| TEXAS INSTRUMENTS INCORPORATED
| Standard Linear and Logic Group
| IBIS Model of SN74ALVC16244A
| 16-BIT BUFFER/DRIVER WITH 3-STATE OUTPUTS
| This file contains package information for the following:
|  TSSOP 48-pin (DGG) package as [Component] ALVC16244A_DGG
|  SSOP 48-pin (DL) package as [Component] ALVC16244A_DL
|  jrBGA 48-pin (GQL) package as [Component] ALVC16244A_GQL
|  jrBGA 48-pin (GQL) package as [Component] ALVC16244A_ZQL
| This device can be powered at the following Vccs:
|  1.8 volt Vcc
|  2.5 volt Vcc
|  2.7 volt Vcc
|  3.3 volt Vcc
| This file provides unique models under the [Model Selector] for each Vcc.
| For operation at a specific Vcc, select the appropriate model after each
| [Model Selector] keyword.
[IBIS Ver]   3.2
[Comment char]  |_char
[File Name]   sn74alvc16244a.ibs
[File Rev]   1.1 | b_die
[Date]   June 26, 2007
[Source]   Data created from TI-SPICE simulations at TI-SLL.
[Notes]   The following is an IBIS list for the SN74ALVC16244A.
   Please contact sllibis@ti.com with questions and
   comments concerning SLL IBIS models.
   This IBIS model is created from a BA (back annotated netlist)
   - FILE REV HISTORY
   - 1.1 Release IBIS file on 05/28/07
[Disclaimer] Property of Texas Instruments Incorporated.  Unauthorized
   reproduction and/or distribution is strictly prohibited.
   This product is protected under copyright law.
   Created  2007, (C) Copyright  2007, Texas Instruments
   Incorporated, All Rights Reserved
   UNLESS THERE IS A SIGNED, WRITTEN AGREEMENT TO THE
   CONTRARY, TEXAS INSTRUMENTS (TI) IS PROVIDING THE IBIS
   MODELS  AND WITHOUT ANY WARRANTY, EXPRESSED OR
   IMPLIED.  TI assumes no liability for:
   1) the accuracy of the IBIS models provided to your
   company;
   2) the proper functioning of these IBIS Models in your
   design or for any resulting applications; or
   3) infringement of patents, copyrights or intellectual
   property rights resulting from your use of these IBIS
   models.
   TI provides IBIS Models as a service to our customers.
   You and your company shall not distribute, sell or give
   these models to anyone else without prior written
   permission from TI.
   TI reserves the right to make changes to our products or
   to discontinue any semiconductor product or service
   without notice, and advises our customers to obtain the
   latest version of relevant information to verify, before
   placing orders, that the information being relied on is
   current.
   Please be aware that your receipt and use of the IBIS
   information provided shall serve as acceptance of these
   terms and conditions.  If you do not accept these terms,
   you should return or destroy the IBIS models and any
   other accompanying information immediately.
| Component SN74ALVC16244A_DGG 48-PIN TSSOP
[Component]   SN74ALVC16244A_DGG
[Manufacturer]   Texas Instruments, Inc.
[Package]
|   typ   min   max
R_pkg   6.200e-02   5.000e-02   7.800e-02
L_pkg   3.527e-09   3.128e-09   4.255e-09
C_pkg   5.300e-13   4.170e-13   6.850e-13
[Pin]   signal_name   model_name   R_pin   L_pin   C_pin
1   N1OE   ALVC16244A_NOE   5.000e-02   4.250e-09   6.710e-13
2   1Y1   ALVC16244A_OUT   5.700e-02   3.956e-09   6.740e-13
3   1Y2   ALVC16244A_OUT   7.100e-02   3.922e-09   6.190e-13
4   GND   GND   7.800e-02   3.841e-09   6.180e-13
5   1Y3   ALVC16244A_OUT   5.600e-02   3.535e-09   5.550e-13
6   1Y4   ALVC16244A_OUT   5.800e-02   3.464e-09   5.030e-13
7   VCC   POWER   6.000e-02   3.362e-09   4.980e-13
8   2Y1   ALVC16244A_OUT   6.100e-02   3.293e-09   4.620e-13
9   2Y2   ALVC16244A_OUT   6.300e-02   3.240e-09   4.550e-13
10   GND   GND   6.300e-02   3.175e-09   4.420e-13
11   2Y3   ALVC16244A_OUT   6.400e-02   3.153e-09   4.290e-13
12   2Y4   ALVC16244A_OUT   6.500e-02   3.128e-09   4.180e-13
13   3Y1   ALVC16244A_OUT   6.500e-02   3.128e-09   4.180e-13
14   3Y2   ALVC16244A_OUT   6.400e-02   3.154e-09   4.290e-13
15   GND   GND   6.300e-02   3.174e-09   4.420e-13
16   3Y3   ALVC16244A_OUT   6.300e-02   3.241e-09   4.550e-13
17   3Y4   ALVC16244A_OUT   6.100e-02   3.293e-09   4.620e-13
18   VCC   POWER   6.000e-02   3.362e-09   4.970e-13
19   4Y1   ALVC16244A_OUT   5.800e-02   3.464e-09   5.030e-13
20   4Y2   ALVC16244A_OUT   5.600e-02   3.537e-09   5.600e-13
21   GND   GND   7.700e-02   3.839e-09   6.260e-13
22   4Y3   ALVC16244A_OUT   7.100e-02   3.917e-09   6.270e-13
23   4Y4   ALVC16244A_OUT   5.800e-02   3.955e-09   6.850e-13
24   N4OE   ALVC16244A_NOE   5.200e-02   4.255e-09   6.790e-13
25   N3OE   ALVC16244A_NOE   5.100e-02   4.254e-09   6.760e-13
26   4A4   ALVC16244A_IN   5.800e-02   3.957e-09   6.790e-13
27   4A3   ALVC16244A_IN   7.100e-02   3.920e-09   6.210e-13
28   GND   GND   7.800e-02   3.843e-09   6.220e-13
29   4A2   ALVC16244A_IN   5.600e-02   3.539e-09   5.600e-13
30   4A1   ALVC16244A_IN   5.800e-02   3.466e-09   5.030e-13
31   VCC   POWER   6.000e-02   3.363e-09   4.970e-13
32   3A4   ALVC16244A_IN   6.100e-02   3.294e-09   4.620e-13
33   3A3   ALVC16244A_IN   6.300e-02   3.241e-09   4.540e-13
34   GND   GND   6.300e-02   3.175e-09   4.410e-13
35   3A2   ALVC16244A_IN   6.400e-02   3.153e-09   4.290e-13
36   3A1   ALVC16244A_IN   6.500e-02   3.129e-09   4.170e-13
37   2A4   ALVC16244A_IN   6.500e-02   3.129e-09   4.170e-13
38   2A3   ALVC16244A_IN   6.400e-02   3.152e-09   4.290e-13
39   GND   GND   6.400e-02   3.176e-09   4.410e-13
40   2A2   ALVC16244A_IN   6.300e-02   3.241e-09   4.540e-13
41   2A1   ALVC16244A_IN   6.100e-02   3.293e-09   4.620e-13
42   VCC   POWER   6.000e-02   3.363e-09   4.970e-13
43   1A4   ALVC16244A_IN   5.800e-02   3.464e-09   5.030e-13
44   1A3   ALVC16244A_IN   5.600e-02   3.534e-09   5.610e-13
45   GND   GND   7.800e-02   3.841e-09   6.260e-13
46   1A2   ALVC16244A_IN   7.100e-02   3.920e-09   6.220e-13
47   1A1   ALVC16244A_IN   5.700e-02   3.955e-09   6.770e-13
48   N2OE   ALVC16244A_NOE   5.100e-02   4.252e-09   6.720e-13
| Component SN74ALVC16244A_DL 48-PIN SSOP
[Component]   SN74ALVC16244A_DL
[Manufacturer]   Texas Instruments, Inc.
[Package]
|   typ   min   max
R_pkg   4.800e-02   3.800e-02   5.300e-02
L_pkg   6.046e-09   5.084e-09   7.968e-09
C_pkg   8.130e-13   5.690e-13   1.157e-12
[Pin]   signal_name   model_name   R_pin   L_pin   C_pin
1   N1OE   ALVC16244A_NOE   4.600e-02   7.968e-09   1.017e-12
2   1Y1   ALVC16244A_OUT   4.400e-02   7.299e-09   1.157e-12
3   1Y2   ALVC16244A_OUT   4.300e-02   6.765e-09   1.058e-12
4   GND   GND   4.100e-02   6.269e-09   9.330e-13
5   1Y3   ALVC16244A_OUT   3.800e-02   5.856e-09   8.290e-13
6   1Y4   ALVC16244A_OUT   4.600e-02   5.802e-09   7.900e-13
7   VCC   POWER   5.000e-02   5.656e-09   7.380e-13
8   2Y1   ALVC16244A_OUT   5.300e-02   5.500e-09   6.430e-13
9   2Y2   ALVC16244A_OUT   5.200e-02   5.304e-09   6.060e-13
10   GND   GND   5.300e-02   5.189e-09   5.830e-13
11   2Y3   ALVC16244A_OUT   5.100e-02   5.084e-09   5.690e-13
12   2Y4   ALVC16244A_OUT   5.300e-02   5.862e-09   8.330e-13
13   3Y1   ALVC16244A_OUT   5.300e-02   5.862e-09   8.330e-13
14   3Y2   ALVC16244A_OUT   5.100e-02   5.084e-09   5.690e-13
15   GND   GND   5.300e-02   5.189e-09   5.830e-13
16   3Y3   ALVC16244A_OUT   5.200e-02   5.304e-09   6.060e-13
17   3Y4   ALVC16244A_OUT   5.300e-02   5.500e-09   6.430e-13
18   VCC   POWER   5.000e-02   5.656e-09   7.380e-13
19   4Y1   ALVC16244A_OUT   4.600e-02   5.802e-09   7.900e-13
20   4Y2   ALVC16244A_OUT   3.800e-02   5.856e-09   8.290e-13
21   GND   GND   4.100e-02   6.269e-09   9.330e-13
22   4Y3   ALVC16244A_OUT   4.300e-02   6.765e-09   1.058e-12
23   4Y4   ALVC16244A_OUT   4.400e-02   7.299e-09   1.157e-12
24   N40E   ALVC16244A_NOE   4.600e-02   7.968e-09   1.017e-12
25   N3OE   ALVC16244A_NOE   4.600e-02   7.968e-09   1.017e-12
26   4A4   ALVC16244A_IN   4.400e-02   7.299e-09   1.157e-12
27   4A3   ALVC16244A_IN   4.300e-02   6.765e-09   1.058e-12
28   GND   GND   4.100e-02   6.269e-09   9.330e-13
29   4A2   ALVC16244A_IN   3.800e-02   5.856e-09   8.290e-13
30   4A1   ALVC16244A_IN   4.600e-02   5.802e-09   7.900e-13
31   VCC   POWER   5.000e-02   5.656e-09   7.380e-13
32   3A4   ALVC16244A_IN   5.300e-02   5.500e-09   6.430e-13
33   3A3   ALVC16244A_IN   5.200e-02   5.304e-09   6.060e-13
34   GND   GND   5.300e-02   5.189e-09   5.830e-13
35   3A2   ALVC16244A_IN   5.100e-02   5.084e-09   5.690e-13
36   3A1   ALVC16244A_IN   5.300e-02   5.862e-09   8.330e-13
37   2A4   ALVC16244A_IN   5.300e-02   5.862e-09   8.330e-13
38   2A3   ALVC16244A_IN   5.100e-02   5.084e-09   5.690e-13
39   GND   GND   5.300e-02   5.189e-09   5.830e-13
40   2A2   ALVC16244A_IN   5.200e-02   5.304e-09   6.060e-13
41   2A1   ALVC16244A_IN   5.300e-02   5.500e-09   6.430e-13
42   VCC   POWER   5.000e-02   5.656e-09   7.380e-13
43   1A4   ALVC16244A_IN   4.600e-02   5.802e-09   7.900e-13
44   1A3   ALVC16244A_IN   3.800e-02   5.856e-09   8.290e-13
45   GND   GND   4.100e-02   6.269e-09   9.330e-13
46   1A2   ALVC16244A_IN   4.300e-02   6.765e-09   1.058e-12
47   1A1   ALVC16244A_IN   4.400e-02   7.299e-09   1.157e-12
48   N2OE   ALVC16244A_NOE   4.600e-02   7.967e-09   1.017e-12
| Component SN74ALVC16244A_GQL 48-PIN JRBGA
[Component]   SN74ALVC16244A_GQL
[Manufacturer]   Texas Instruments, Inc.
[Package]
|   typ   min   max
R_pkg   7.900e-02   4.500e-02   9.400e-02
L_pkg   2.264e-09   1.398e-09   2.722e-09
C_pkg   3.060e-13   1.170e-13   4.040e-13
[Pin]   signal_name   model_name   R_pin   L_pin   C_pin
A1   N1OE   ALVC16244A_NOE   5.100e-02   1.531e-09   2.100e-13
B2   1Y1   ALVC16244A_OUT   7.300e-02   2.572e-09   3.120e-13
B1   1Y2   ALVC16244A_OUT   7.100e-02   1.835e-09   2.320e-13
B3   GND   GND   9.400e-02   2.717e-09   3.830e-13
C2   1Y3   ALVC16244A_OUT   8.900e-02   2.534e-09   3.500e-13
C1   1Y4   ALVC16244A_OUT   7.100e-02   1.831e-09   2.310e-13
C3   VCC   POWER   9.400e-02   2.722e-09   3.920e-13
D2   2Y1   ALVC16244A_OUT   9.000e-02   2.551e-09   3.520e-13
D1   2Y2   ALVC16244A_OUT   7.200e-02   1.846e-09   2.440e-13
D3   GND   GND   9.400e-02   2.719e-09   4.030e-13
E2   2Y3   ALVC16244A_OUT   8.900e-02   2.541e-09   3.510e-13
E1   2Y4   ALVC16244A_OUT   7.200e-02   1.850e-09   2.270e-13
F1   3Y1   ALVC16244A_OUT   7.200e-02   1.850e-09   2.270e-13
F2   3Y2   ALVC16244A_OUT   8.900e-02   2.541e-09   3.510e-13
G3   GND   GND   9.400e-02   2.718e-09   4.040e-13
G1   3Y3   ALVC16244A_OUT   7.200e-02   1.847e-09   2.440e-13
G2   3Y4   ALVC16244A_OUT   9.000e-02   2.551e-09   3.520e-13
H3   VCC   POWER   9.400e-02   2.721e-09   3.920e-13
H1   4Y1   ALVC16244A_OUT   7.000e-02   1.830e-09   2.310e-13
H2   4Y2   ALVC16244A_OUT   8.800e-02   2.524e-09   3.500e-13
J3   GND   GND   9.300e-02   2.709e-09   3.820e-13
J1   4Y3   ALVC16244A_OUT   7.100e-02   1.851e-09   2.330e-13
J2   4Y4   ALVC16244A_OUT   5.600e-02   2.605e-09   3.900e-13
K1   N4OE   ALVC16244A_NOE   4.500e-02   1.398e-09   1.170e-13
K6   N3OE   ALVC16244A_NOE   4.500e-02   1.512e-09   1.930e-13
J5   4A4   ALVC16244A_IN   5.500e-02   2.492e-09   3.130e-13
J6   4A3   ALVC16244A_IN   7.000e-02   1.821e-09   2.300e-13
J4   GND   GND   9.300e-02   2.703e-09   3.820e-13
H5   4A2   ALVC16244A_IN   8.900e-02   2.529e-09   3.500e-13
H6   4A1   ALVC16244A_IN   7.100e-02   1.826e-09   2.300e-13
H4   VCC   POWER   9.400e-02   2.722e-09   3.910e-13
G5   3A4   ALVC16244A_IN   9.000e-02   2.551e-09   3.520e-13
G6   3A3   ALVC16244A_IN   7.200e-02   1.846e-09   2.440e-13
G4   GND   GND   9.400e-02   2.719e-09   4.040e-13
F5   3A2   ALVC16244A_IN   8.800e-02   2.510e-09   3.490e-13
F6   3A1   ALVC16244A_IN   7.200e-02   1.850e-09   2.270e-13
E6   2A4   ALVC16244A_IN   7.100e-02   1.850e-09   2.270e-13
E5   2A3   ALVC16244A_IN   8.900e-02   2.529e-09   3.500e-13
D4   GND   GND   9.400e-02   2.719e-09   4.030e-13
D6   2A2   ALVC16244A_IN   7.200e-02   1.847e-09   2.430e-13
D5   2A1   ALVC16244A_IN   8.900e-02   2.550e-09   3.520e-13
C4   VCC   POWER   9.400e-02   2.722e-09   3.910e-13
C6   1A4   ALVC16244A_IN   7.100e-02   1.827e-09   2.300e-13
C5   1A3   ALVC16244A_IN   8.900e-02   2.539e-09   3.500e-13
B4   GND   GND   9.300e-02   2.705e-09   3.820e-13
B6   1A2   ALVC16244A_IN   7.100e-02   1.831e-09   2.270e-13
B5   1A1   ALVC16244A_IN   7.300e-02   2.685e-09   3.800e-13
A6   N2OE   ALVC16244A_NOE   5.100e-02   1.417e-09   1.330e-13
| Component SN74ALVC16244A_ZQL 48-PIN JRBGA
[Component]   SN74ALVC16244A_ZQL
[Manufacturer]   Texas Instruments, Inc.
[Package]
|   typ   min   max
R_pkg   7.900e-02   4.500e-02   9.400e-02
L_pkg   2.264e-09   1.398e-09   2.722e-09
C_pkg   3.060e-13   1.170e-13   4.040e-13
[Pin]   signal_name   model_name   R_pin   L_pin   C_pin
A1   N1OE   ALVC16244A_NOE   5.100e-02   1.531e-09   2.100e-13
B2   1Y1   ALVC16244A_OUT   7.300e-02   2.572e-09   3.120e-13
B1   1Y2   ALVC16244A_OUT   7.100e-02   1.835e-09   2.320e-13
B3   GND   GND   9.400e-02   2.717e-09   3.830e-13
C2   1Y3   ALVC16244A_OUT   8.900e-02   2.534e-09   3.500e-13
C1   1Y4   ALVC16244A_OUT   7.100e-02   1.831e-09   2.310e-13
C3   VCC   POWER   9.400e-02   2.722e-09   3.920e-13
D2   2Y1   ALVC16244A_OUT   9.000e-02   2.551e-09   3.520e-13
D1   2Y2   ALVC16244A_OUT   7.200e-02   1.846e-09   2.440e-13
D3   GND   GND   9.400e-02   2.719e-09   4.030e-13
E2   2Y3   ALVC16244A_OUT   8.900e-02   2.541e-09   3.510e-13
E1   2Y4   ALVC16244A_OUT   7.200e-02   1.850e-09   2.270e-13
F1   3Y1   ALVC16244A_OUT   7.200e-02   1.850e-09   2.270e-13
F2   3Y2   ALVC16244A_OUT   8.900e-02   2.541e-09   3.510e-13
G3   GND   GND   9.400e-02   2.718e-09   4.040e-13
G1   3Y3   ALVC16244A_OUT   7.200e-02   1.847e-09   2.440e-13
G2   3Y4   ALVC16244A_OUT   9.000e-02   2.551e-09   3.520e-13
H3   VCC   POWER   9.400e-02   2.721e-09   3.920e-13
H1   4Y1   ALVC16244A_OUT   7.000e-02   1.830e-09   2.310e-13
H2   4Y2   ALVC16244A_OUT   8.800e-02   2.524e-09   3.500e-13
J3   GND   GND   9.300e-02   2.709e-09   3.820e-13
J1   4Y3   ALVC16244A_OUT   7.100e-02   1.851e-09   2.330e-13
J2   4Y4   ALVC16244A_OUT   5.600e-02   2.605e-09   3.900e-13
K1   N4OE   ALVC16244A_NOE   4.500e-02   1.398e-09   1.170e-13
K6   N3OE   ALVC16244A_NOE   4.500e-02   1.512e-09   1.930e-13
J5   4A4   ALVC16244A_IN   5.500e-02   2.492e-09   3.130e-13
J6   4A3   ALVC16244A_IN   7.000e-02   1.821e-09   2.300e-13
J4   GND   GND   9.300e-02   2.703e-09   3.820e-13
H5   4A2   ALVC16244A_IN   8.900e-02   2.529e-09   3.500e-13
H6   4A1   ALVC16244A_IN   7.100e-02   1.826e-09   2.300e-13
H4   VCC   POWER   9.400e-02   2.722e-09   3.910e-13
G5   3A4   ALVC16244A_IN   9.000e-02   2.551e-09   3.520e-13
G6   3A3   ALVC16244A_IN   7.200e-02   1.846e-09   2.440e-13
G4   GND   GND   9.400e-02   2.719e-09   4.040e-13
F5   3A2   ALVC16244A_IN   8.800e-02   2.510e-09   3.490e-13
F6   3A1   ALVC16244A_IN   7.200e-02   1.850e-09   2.270e-13
E6   2A4   ALVC16244A_IN   7.100e-02   1.850e-09   2.270e-13
E5   2A3   ALVC16244A_IN   8.900e-02   2.529e-09   3.500e-13
D4   GND   GND   9.400e-02   2.719e-09   4.030e-13
D6   2A2   ALVC16244A_IN   7.200e-02   1.847e-09   2.430e-13
D5   2A1   ALVC16244A_IN   8.900e-02   2.550e-09   3.520e-13
C4   VCC   POWER   9.400e-02   2.722e-09   3.910e-13
C6   1A4   ALVC16244A_IN   7.100e-02   1.827e-09   2.300e-13
C5   1A3   ALVC16244A_IN   8.900e-02   2.539e-09   3.500e-13
B4   GND   GND   9.300e-02   2.705e-09   3.820e-13
B6   1A2   ALVC16244A_IN   7.100e-02   1.831e-09   2.270e-13
B5   1A1   ALVC16244A_IN   7.300e-02   2.685e-09   3.800e-13
A6   N2OE   ALVC16244A_NOE   5.100e-02   1.417e-09   1.330e-13
| Model ALVC16244A_NOE
[Model Selector]   ALVC16244A_NOE
ALVC16244A_NOE_18   1.8 volt Vcc
ALVC16244A_NOE_25   2.5 volt Vcc
ALVC16244A_NOE_27   2.7 volt Vcc
ALVC16244A_NOE_33   3.3 volt Vcc
| Model ALVC16244A_IN
[Model Selector]   ALVC16244A_IN
ALVC16244A_IN_18   1.8 volt Vcc
ALVC16244A_IN_25   2.5 volt Vcc
ALVC16244A_IN_27   2.7 volt Vcc
ALVC16244A_IN_33   3.3 volt Vcc
| Model ALVC16244A_OUT
[Model Selector]   ALVC16244A_OUT
ALVC16244A_OUT_18   1.8 volt Vcc
ALVC16244A_OUT_25   2.5 volt Vcc
ALVC16244A_OUT_27   2.7 volt Vcc
ALVC16244A_OUT_33   3.3 volt Vcc
| Models and submodels in the file (12): ALVC16244A_NOE_18 (Input), ALVC16244A_NOE_25 (Input), ALVC16244A_NOE_27 (Input), ALVC16244A_NOE_33 (Input), ALVC16244A_IN_18 (Input), ALVC16244A_IN_25 (Input), ALVC16244A_IN_27 (Input), ALVC16244A_IN_33 (Input), ALVC16244A_OUT_18 (3-state), ALVC16244A_OUT_25 (3-state), ALVC16244A_OUT_27 (3-state), ALVC16244A_OUT_33 (3-state)
